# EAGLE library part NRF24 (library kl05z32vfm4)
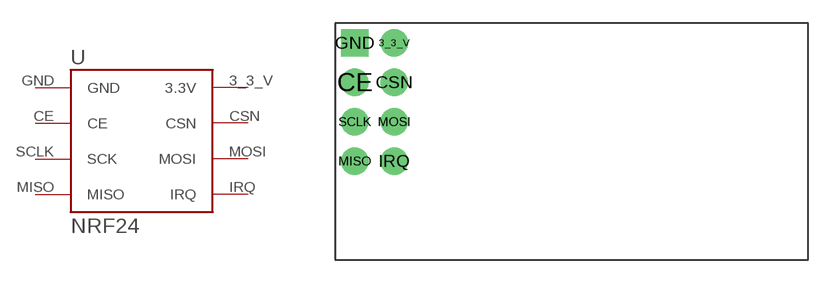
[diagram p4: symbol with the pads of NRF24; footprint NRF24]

Designator prefix -

## NRF24  [NRF24]
3_3_V  3.3V
CE  CE
CSN  CSN
GND  GND
IRQ  IRQ
MISO  MISO
MOSI  MOSI
SCLK  SCK

## Footprint NRF24 (pad centres in mm)
drill 0.9 pad 1.778: 3_3_V 3.81,13.97; CE 1.27,11.43; CSN 3.81,11.43; IRQ 3.81,6.35; MISO 1.27,6.35; MOSI 3.81,8.89; SCLK 1.27,8.89
drill 0.9 pad 1.778 square: GND 1.27,13.97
